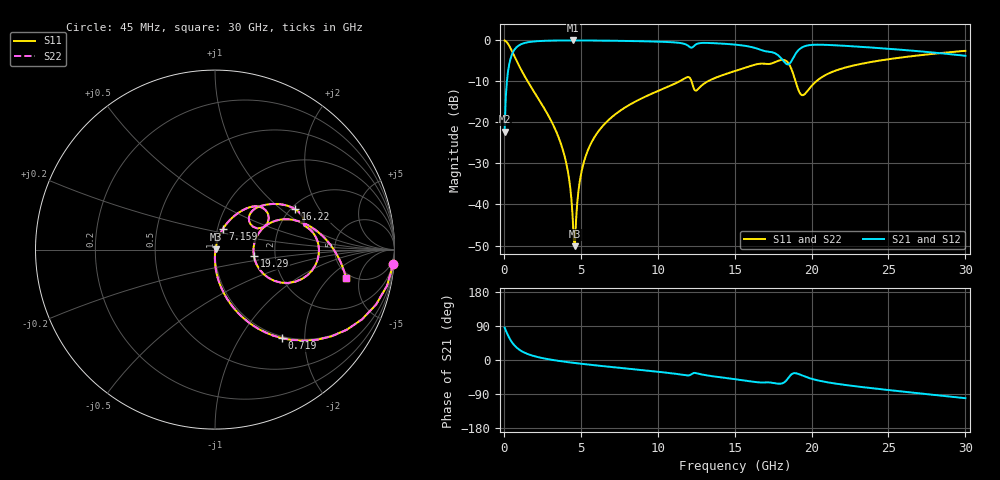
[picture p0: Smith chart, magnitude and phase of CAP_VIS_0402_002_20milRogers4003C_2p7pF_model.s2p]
! S-parameter model data by Modelithics Inc.  support@modelithics.com  813-866-6335  Tampa FL USA
! S-Parameter data specifications:
! Substrate: 20-mil Rogers 4003C, substrate thickness, H=0.508mm, Dielectric constant, Er=3.75
! PCB Mounting Pad Footprint: Pad width, PadW=0.50mm , Pad length, PadL=0.50mm , Pad gap, PadG (edge-to-edge)=0.40mm , Reference planes=1.4mm apart
! Created Wed Nov 18 12:45:53 2015
# hz S ma R 50
! 2 Port Network Data from SP1.SP block
! freq  magS11  angS11  magS21  angS21  magS12  angS12  magS22  angS22
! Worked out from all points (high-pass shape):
!   401 points, 45 MHz to 30 GHz, reference 50 ohm
!   highest |S21| = -0.02 dB at 4.463 GHz (marker M1); lowest = -22.2 dB at 45 MHz (marker M2)
!   |S21| within 3 dB of the highest: 571 MHz to 17.54 GHz (16.97 GHz wide, 187 % of centre); 19.01 GHz to 28.08 GHz (9.07 GHz wide, 38.5 % of centre)
!   lowest |S11| = -50.2 dB at 4.613 GHz (marker M3), VSWR 1.01, Z = 50.3 + j0.124 ohm
!   |S11| at or under -10 dB: 1.546 GHz to 11.41 GHz (9.863 GHz wide, 152 % of centre); 12.2 GHz to 13.24 GHz (1.046 GHz wide, 8.22 % of centre); 18.96 GHz to 20.3 GHz (1.34 GHz wide, 6.82 % of centre)
!   |S22| runs from -50.2 to 0.0 dB; largest |S21 - S12| = 0
!   S11 on the Smith chart (normalised r, x): 45 MHz: 1, -25; 719 MHz: 0.97, -1.55; 7.159 GHz: 1.06, +0.25; 16.22 GHz: 2.09, +1.26; 19.29 GHz: 1.55, -0.12; 30 GHz: 4.55, -3.20
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4.5e7  0.997 -4.5  0.07725 85.5  0.07725 85.5  0.997 -4.5
3.4455e8  0.8586 -31.4  0.5122 58.6  0.5122 58.6  0.8586 -31.4
7.189875e8  0.6187 -52.9  0.7847 37.0  0.7847 37.0  0.6187 -52.9
1.617638e9  0.3002 -75.0  0.9523 14.7  0.9523 14.7  0.3002 -75.0
3.6396e9  0.05962 -90.5  0.9958 -2.8  0.9958 -2.8  0.05962 -90.5
4.163812e9  0.02492 -89.9  0.9971 -5.7  0.9971 -5.7  0.02492 -89.9
4.463362e9  0.007378 -76.6  0.9972 -7.2  0.9972 -7.2  0.007378 -76.6
4.613138e9  0.003104 23.4  0.9972 -7.9  0.9972 -7.9  0.003104 23.4
5.062462e9  0.02593 73.7  0.9967 -10.1  0.9967 -10.1  0.02593 73.7
5.811338e9  0.06263 73.7  0.9948 -13.5  0.9948 -13.5  0.06263 73.7
7.159312e9  0.1222 69.2  0.9888 -19.2  0.9888 -19.2  0.1222 69.2
1.007992e10  0.2444 57.3  0.9636 -31.3  0.9636 -31.3  0.2444 57.3
1.195211e10  0.3575 37.7  0.8654 -40.9  0.8654 -40.9  0.3575 37.7
1.255121e10  0.2474 39.7  0.9063 -35.2  0.9063 -35.2  0.2474 39.7
1.50225e10  0.4233 36.9  0.8876 -50.6  0.8876 -50.6  0.4233 36.9
1.62207e10  0.4993 26.9  0.8185 -57.5  0.8185 -57.5  0.4993 26.9
1.831755e10  0.5664 -8.8  0.5234 -55.8  0.5234 -55.8  0.5664 -8.8
1.876688e10  0.4105 -26.6  0.592 -35.9  0.592 -35.9  0.4105 -26.6
1.929109e10  0.2204 -9.9  0.8014 -39.2  0.8014 -39.2  0.2204 -9.9
2.003996e10  0.2832 23.3  0.8809 -50.1  0.8809 -50.1  0.2832 23.3
2.505742e10  0.591 8.7  0.7882 -79.5  0.7882 -79.5  0.591 8.7
3e10  0.746 -12.1  0.6485 -100.8  0.6485 -100.8  0.746 -12.1
